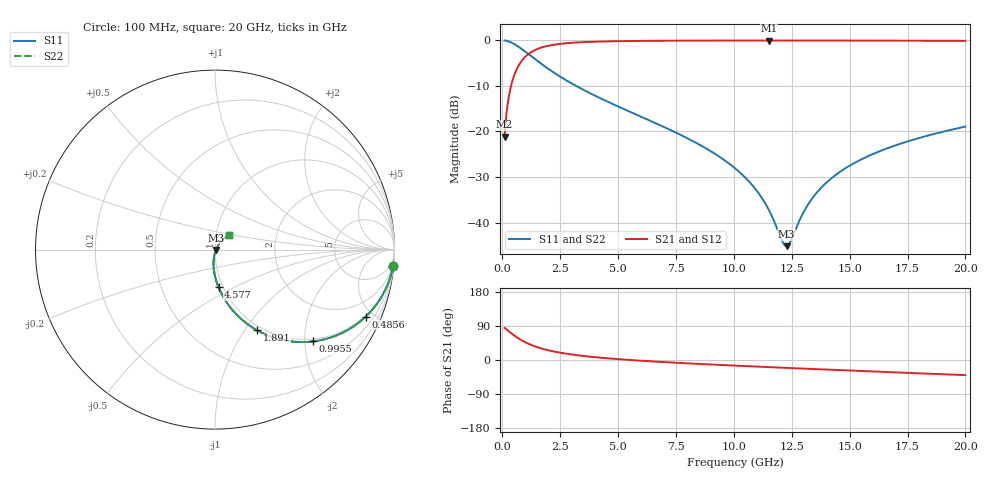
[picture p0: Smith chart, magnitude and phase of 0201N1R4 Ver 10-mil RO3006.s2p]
# GHz S MA R 50
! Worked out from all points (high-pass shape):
!   1601 points, 100 MHz to 20 GHz, reference 50 ohm
!   highest |S21| = -0.05 dB at 11.52 GHz (marker M1); lowest = -21.1 dB at 100 MHz (marker M2)
!   |S21| within 3 dB of the highest: 1.121 GHz to end of sweep
!   lowest |S11| = -45.2 dB at 12.28 GHz (marker M3), VSWR 1.01, Z = 50.5 - j0.195 ohm
!   |S11| at or under -10 dB: 3.186 GHz to end of sweep
!   |S22| runs from -45.2 to 0.0 dB; largest |S21 - S12| = 0
!   S11 on the Smith chart (normalised r, x): 100 MHz: 1, -22; 485.6 MHz: 0.94, -4.52; 995.5 MHz: 0.94, -2.19; 1.891 GHz: 0.94, -1.14; 4.577 GHz: 0.95, -0.42; 20 GHz: 1.15, +0.19
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0.1  0.9961 -5.2  0.08766 84.8  0.08766 84.8  0.9961 -5.2
0.299  0.9669 -15.3  0.2545 74.7  0.2545 74.7  0.9669 -15.3
0.4855625  0.919 -24.0  0.3932 66.0  0.3932 66.0  0.919 -24.0
0.7094375  0.8469 -33.2  0.5303 56.7  0.5303 56.7  0.8469 -33.2
0.9955  0.7493 -43.0  0.6604 46.8  0.6604 46.8  0.7493 -43.0
1.418375  0.6195 -53.9  0.7828 35.9  0.7828 35.9  0.6195 -53.9
1.891  0.5056 -62.6  0.8601 27.1  0.8601 27.1  0.5056 -62.6
3.420812  0.2938 -78.1  0.9524 11.2  0.9524 11.2  0.2938 -78.1
4.5775  0.2106 -84.6  0.9737 4.3  0.9737 4.3  0.2106 -84.6
6.741625  0.1194 -92.5  0.9883 -4.6  0.9883 -4.6  0.1194 -92.5
8.70675  0.06726 -96.9  0.9927 -11.0  0.9927 -11.0  0.06726 -96.9
10.05  0.03944 -97.4  0.9939 -14.8  0.9939 -14.8  0.03944 -97.4
10.88331  0.02423 -94.6  0.9942 -17.1  0.9942 -17.1  0.02423 -94.6
11.51763  0.01368 -85.7  0.9943 -18.8  0.9943 -18.8  0.01368 -85.7
12.08975  0.006255 -49.2  0.9942 -20.3  0.9942 -20.3  0.006255 -49.2
12.27631  0.005514 -20.5  0.9942 -20.8  0.9942 -20.8  0.005514 -20.5
12.438  0.00614 4.2  0.9941 -21.2  0.9941 -21.2  0.00614 4.2
12.94794  0.01213 39.8  0.994 -22.6  0.994 -22.6  0.01213 39.8
13.37081  0.01822 48.1  0.9938 -23.6  0.9938 -23.6  0.01822 48.1
14.67675  0.0374 53.9  0.993 -26.9  0.993 -26.9  0.0374 53.9
16.69162  0.06628 52.6  0.9911 -31.9  0.9911 -31.9  0.06628 52.6
20  0.113 46.5  0.9862 -40.0  0.9862 -40.0  0.113 46.5
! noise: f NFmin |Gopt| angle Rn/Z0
0.1  0.0009786  0.9583  0.8011  0.005291
2.301  0.00536  0.8262  4.438  0.006473
4.515  0.008286  0.7844  8.088  0.007858
6.729  0.01081  0.7577  11.75  0.008935
8.943  0.01311  0.7382  15.39  0.00985
11.14  0.01527  0.7232  18.98  0.01066
13.36  0.01735  0.7112  22.56  0.01139
15.57  0.01936  0.7014  26.1  0.01208
17.79  0.02134  0.6936  29.6  0.01272
20  0.02329  0.6872  33.05  0.01334
